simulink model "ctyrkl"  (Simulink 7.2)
settings: Solver=ode45  StartTime=0.0  StopTime=10.0  MaxStep=0.05  RelTol=1e-3
InitFcn:
  | init_ctyrkloub;
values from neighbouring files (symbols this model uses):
  L1 = 3    [init_ctyrkloub.m]    (also in init_klik.m = 1.5; init_withworth.m = 2)
  L2 = 5    [init_ctyrkloub.m]    (also in init_klik.m = v/sin(uhel3); init_withworth.m)
  L3 = 0.5    [init_ctyrkloub.m]    (also in init_klik.m = L1/(sin(uhel1)))
  L4 = 1    [init_ctyrkloub.m]
  omega = 1    [init_ctyrkloub.m]    (also in init_klik.m = 5; init_withworth.m = 0.5)
undefined symbols (not defined in the file or in its folder): deg, kg, m, N, rad, s
libraries: mblibv1 x17, simulink x3

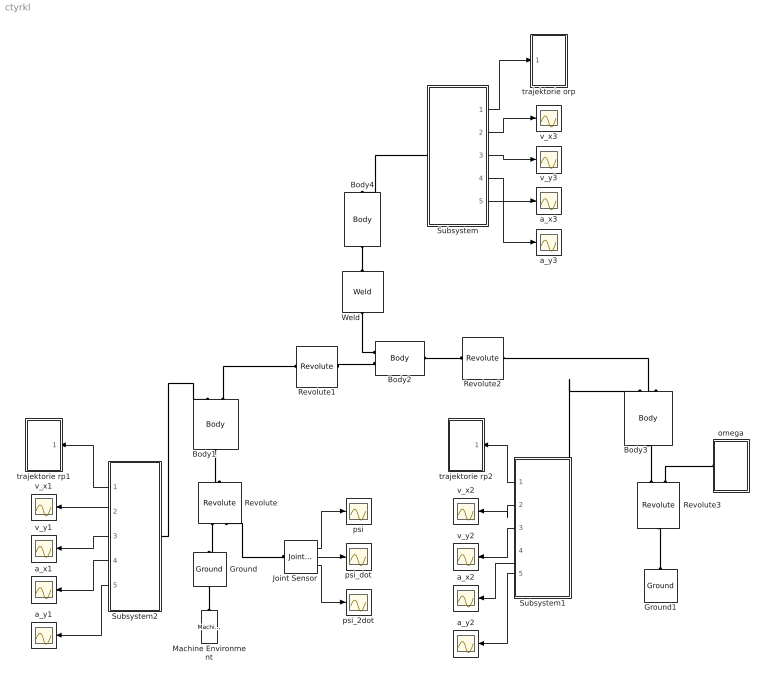
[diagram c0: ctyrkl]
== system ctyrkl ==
  Body1 : mblibv1/Bodies/Body  Orientation=up  DialogController=MECH.DynMechDlgSource  PhysicalDomain=mechanical  SubClassName=Unknown  LeftPortType=workingframe  RightPortType=workingframe  LConnTagsString=CS1  RConnTagsString=CS3|CS2  UpdateFromCAD=off  DialogClass=MechanicalBodyBlock  Mass=1  MassUnits=kg  InertiaUnits=kg*m^2  Inertia=eye(3)  Shape=Cylinder  ShapeDims=[1 1]  ShapeUnits=m  ShapeUse=false  Density=1  DensityUnits=kg/m^3  DensityUse=false  GraphicsMode=MACHINE_DEFAULT  BodyColorSelMode=MACHINE_DEFAULT  BodyColor=[1 0 0]  AttachedToCS=CG  CG=Left$CG$[L1*cos(pi/3) L1*sin(pi/3) 0]/2$CS1$CS1$m$[0 0 0]$Euler X-Y-Z$deg$WORLD$false$none  WorkingFrames=Right$CS3$[0 0 0]$CS2$CS2$m$[0 0 0]$Euler X-Y-Z$deg$WORLD$true$none#Left$CS1$[0 0 0]$Adjoining$Adjoining$m$[0 0 0]$Euler X-Y-Z$deg$WORLD$true$none#Right$CS2$[L1*cos(pi/3) L1*sin(pi/3) 0]$CS1$CS1$m$[0 0 0]$Euler X-Y-Z$deg$WORLD$true$none  CGPos=[L1*cos(pi/3) L1*sin(pi/3) 0]/2  CGRot=[0 0 0]  CS0Pos=[]  CS0Rot=[]  CS1Pos=[0 0 0]  CS1Rot=[0 0 0]  CS2Pos=[L1*cos(pi/3) L1*sin(pi/3) 0]  CS2Rot=[0 0 0]  CS3Pos=[0 0 0]  CS3Rot=[0 0 0]  CS4Pos=[]  CS4Rot=[]  CS5Pos=[]  CS5Rot=[]  CS6Pos=[]  CS6Rot=[]  CS7Pos=[]  CS7Rot=[]  CS8Pos=[]  CS8Rot=[]  CS9Pos=[]  CS9Rot=[]  CS10Pos=[]  CS10Rot=[]  CS11Pos=[]  CS11Rot=[]  CS12Pos=[]  CS12Rot=[]  CS13Pos=[]  CS13Rot=[]  CS14Pos=[]  CS14Rot=[]  CS15Pos=[]  CS15Rot=[]  CS16Pos=[]  CS16Rot=[]  CS17Pos=[]  CS17Rot=[]  CS18Pos=[]  CS18Rot=[]  CS19Pos=[]  CS19Rot=[]  CS20Pos=[]  CS20Rot=[]
  Body2 : mblibv1/Bodies/Body  DialogController=MECH.DynMechDlgSource  PhysicalDomain=mechanical  SubClassName=Unknown  LeftPortType=workingframe  RightPortType=workingframe  LConnTagsString=CG|CS1  RConnTagsString=CS2  UpdateFromCAD=off  DialogClass=MechanicalBodyBlock  Mass=1  MassUnits=kg  InertiaUnits=kg*m^2  Inertia=eye(3)  Shape=Cylinder  ShapeDims=[1 1]  ShapeUnits=m  ShapeUse=false  Density=1  DensityUnits=kg/m^3  DensityUse=false  GraphicsMode=MACHINE_DEFAULT  BodyColorSelMode=MACHINE_DEFAULT  BodyColor=[1 0 0]  AttachedToCS=CG  CG=Left$CG$[L2*cos(pi/6) -L2*sin(pi/6) 0]/2$CS1$CS1$m$[0 0 0]$Euler X-Y-Z$deg$WORLD$true$none  WorkingFrames=Left$CS1$[0 0 0]$Adjoining$Adjoining$m$[0 0 0]$Euler X-Y-Z$deg$WORLD$true$none#Right$CS2$[L2*cos(pi/6) -L2*sin(pi/6) 0]$CS1$CS1$m$[0 0 0]$Euler X-Y-Z$deg$WORLD$true$none  CGPos=[L2*cos(pi/6) -L2*sin(pi/6) 0]/2  CGRot=[0 0 0]  CS0Pos=[]  CS0Rot=[]  CS1Pos=[0 0 0]  CS1Rot=[0 0 0]  CS2Pos=[L2*cos(pi/6) -L2*sin(pi/6) 0]  CS2Rot=[0 0 0]  CS3Pos=[]  CS3Rot=[]  CS4Pos=[]  CS4Rot=[]  CS5Pos=[]  CS5Rot=[]  CS6Pos=[]  CS6Rot=[]  CS7Pos=[]  CS7Rot=[]  CS8Pos=[]  CS8Rot=[]  CS9Pos=[]  CS9Rot=[]  CS10Pos=[]  CS10Rot=[]  CS11Pos=[]  CS11Rot=[]  CS12Pos=[]  CS12Rot=[]  CS13Pos=[]  CS13Rot=[]  CS14Pos=[]  CS14Rot=[]  CS15Pos=[]  CS15Rot=[]  CS16Pos=[]  CS16Rot=[]  CS17Pos=[]  CS17Rot=[]  CS18Pos=[]  CS18Rot=[]  CS19Pos=[]  CS19Rot=[]  CS20Pos=[]  CS20Rot=[]
  Body3 : mblibv1/Bodies/Body  Orientation=down  DialogController=MECH.DynMechDlgSource  PhysicalDomain=mechanical  SubClassName=Unknown  LeftPortType=workingframe  RightPortType=workingframe  LConnTagsString=CS3|CS1  RConnTagsString=CS2  UpdateFromCAD=off  DialogClass=MechanicalBodyBlock  Mass=1  MassUnits=kg  InertiaUnits=kg*m^2  Inertia=eye(3)  Shape=Cylinder  ShapeDims=[1 1]  ShapeUnits=m  ShapeUse=false  Density=1  DensityUnits=kg/m^3  DensityUse=false  GraphicsMode=MACHINE_DEFAULT  BodyColorSelMode=MACHINE_DEFAULT  BodyColor=[1 0 0]  AttachedToCS=CG  CG=Left$CG$[L3*sin(pi/4) -L3*cos(pi/4) 0]/2$CS1$CS1$m$[0 0 0]$Euler X-Y-Z$deg$WORLD$false$none  WorkingFrames=Left$CS3$[0 0 0]$CS1$CS1$m$[0 0 0]$Euler X-Y-Z$deg$WORLD$true$none#Left$CS1$[0 0 0]$Adjoining$Adjoining$m$[0 0 0]$Euler X-Y-Z$deg$WORLD$true$none#Right$CS2$[L3*sin(pi/4) -L3*cos(pi/4) 0]$CS1$CS1$m$[0 0 0]$Euler X-Y-Z$deg$WORLD$true$none  CGPos=[L3*sin(pi/4) -L3*cos(pi/4) 0]/2  CGRot=[0 0 0]  CS0Pos=[]  CS0Rot=[]  CS1Pos=[0 0 0]  CS1Rot=[0 0 0]  CS2Pos=[L3*sin(pi/4) -L3*cos(pi/4) 0]  CS2Rot=[0 0 0]  CS3Pos=[0 0 0]  CS3Rot=[0 0 0]  CS4Pos=[]  CS4Rot=[]  CS5Pos=[]  CS5Rot=[]  CS6Pos=[]  CS6Rot=[]  CS7Pos=[]  CS7Rot=[]  CS8Pos=[]  CS8Rot=[]  CS9Pos=[]  CS9Rot=[]  CS10Pos=[]  CS10Rot=[]  CS11Pos=[]  CS11Rot=[]  CS12Pos=[]  CS12Rot=[]  CS13Pos=[]  CS13Rot=[]  CS14Pos=[]  CS14Rot=[]  CS15Pos=[]  CS15Rot=[]  CS16Pos=[]  CS16Rot=[]  CS17Pos=[]  CS17Rot=[]  CS18Pos=[]  CS18Rot=[]  CS19Pos=[]  CS19Rot=[]  CS20Pos=[]  CS20Rot=[]
  Body4 : mblibv1/Bodies/Body  Orientation=up  DialogController=MECH.DynMechDlgSource  PhysicalDomain=mechanical  SubClassName=Unknown  LeftPortType=workingframe  RightPortType=workingframe  LConnTagsString=CS1  RConnTagsString=CS2  UpdateFromCAD=off  DialogClass=MechanicalBodyBlock  Mass=1  MassUnits=kg  InertiaUnits=kg*m^2  Inertia=eye(3)  Shape=Cylinder  ShapeDims=[1 1]  ShapeUnits=m  ShapeUse=false  Density=1  DensityUnits=kg/m^3  DensityUse=false  GraphicsMode=MACHINE_DEFAULT  BodyColorSelMode=MACHINE_DEFAULT  BodyColor=[1 0 0]  AttachedToCS=CG  CG=Left$CG$[0 L4 0]/2$CS1$CS1$m$[0 0 0]$Euler X-Y-Z$deg$WORLD$false$none  WorkingFrames=Left$CS1$[0 0 0]$Adjoining$Adjoining$m$[0 0 0]$Euler X-Y-Z$deg$WORLD$true$none#Right$CS2$[0 L4 0]$CS1$CS1$m$[0 0 0]$Euler X-Y-Z$deg$WORLD$true$none  CGPos=[0 L4 0]/2  CGRot=[0 0 0]  CS0Pos=[]  CS0Rot=[]  CS1Pos=[0 0 0]  CS1Rot=[0 0 0]  CS2Pos=[0 L4 0]  CS2Rot=[0 0 0]  CS3Pos=[]  CS3Rot=[]  CS4Pos=[]  CS4Rot=[]  CS5Pos=[]  CS5Rot=[]  CS6Pos=[]  CS6Rot=[]  CS7Pos=[]  CS7Rot=[]  CS8Pos=[]  CS8Rot=[]  CS9Pos=[]  CS9Rot=[]  CS10Pos=[]  CS10Rot=[]  CS11Pos=[]  CS11Rot=[]  CS12Pos=[]  CS12Rot=[]  CS13Pos=[]  CS13Rot=[]  CS14Pos=[]  CS14Rot=[]  CS15Pos=[]  CS15Rot=[]  CS16Pos=[]  CS16Rot=[]  CS17Pos=[]  CS17Rot=[]  CS18Pos=[]  CS18Rot=[]  CS19Pos=[]  CS19Rot=[]  CS20Pos=[]  CS20Rot=[]
  Ground : mblibv1/Bodies/Ground  Orientation=up  DialogController=MECH.DynMechDlgSource  SystemSampleTime=-1  UpdateFromCAD=off  LeftPortType=env  RightPortType=workingframe  PhysicalDomain=Mechanical  DialogClass=GroundBlock  CoordPosition=[0 0 0]  CoordPositionUnits=m  StateVectorMgrId=0  MachineId=[1 0]  ShowEnvPort=on
  Ground1 : mblibv1/Bodies/Ground  Orientation=up  DialogController=MECH.DynMechDlgSource  SystemSampleTime=-1  UpdateFromCAD=off  LeftPortType=env  RightPortType=workingframe  PhysicalDomain=Mechanical  DialogClass=GroundBlock  CoordPosition=[L1*cos(pi/3)+L2*cos(pi/6)+L3*sin(pi/4) L1*sin(pi/3)-L2*sin(pi/6)-L3*cos(pi/4) 0]  CoordPositionUnits=m  StateVectorMgrId=-1  MachineId=[0 0]  ShowEnvPort=off
  Joint Sensor : mblibv1/Sensors &  Actuators/Joint Sensor  DialogController=MECH.DynMechDlgSource  SystemSampleTime=-1  UpdateFromCAD=off  PhysicalDomain=Mechanical  PortType=blob  Muxed=off  Pose=off  Angle=on  AngleUnits=rad  ArcVelocity=on  ArcVelocityUnits=rad/s  ArcAcceleration=on  ArcAccelerationUnits=rad/s^2  CoordPosition=on  CoordPositionUnits=m  Velocity=off  VelocityUnits=m/s  Acceleration=off  AccelerationUnits=m/s^2  Quaternion=on  QuaternionDT=off  QuaternionDDT=off  QuaternionUnits=off  OutputVector=[1]  ActiveIO=on  Width=3  DialogClass=MechanicalSensorBlock  Primitive=R1  Force=off  ForceUnits=N  Torque=off  TorqueUnits=N*m  ReferenceFrame=Absolute (World)  ReactionSensedSide=Base  ReactionReferenceFrame=Absolute (World)  ReactionForce=off  ReactionForceUnits=N  ReactionMoment=off  ReactionMomentUnits=N*m
  Machine Environment : mblibv1/Bodies/Machine Environment  Orientation=up  DialogController=MECH.DialogSource  SystemSampleTime=-1  PortType=env  PhysicalDomain=Mechanical  DialogTemplateClass=MECH.MachineEnvironment  SyncWhenCopied=off  Gravity=[0 -9.81 0]  GravityUnits=m/s^2  GravityAsSignal=off  Dimensionality=Auto-detect  AnalysisType=Kinematics  LinearAssemblyTolerance=1e-3  LinearAssemblyToleranceUnits=m  AngularAssemblyTolerance=1e-3  AngularAssemblyToleranceUnits=rad  ConstraintSolverType=Stabilizing  ConstraintRelTolerance=1e-4  ConstraintAbsTolerance=1e-4  UseRobustSingularityHandling=off  RedundancyAnalysisToleranceType=Automatically select tolerance  RedundancyAnalysisTolerance=1e-14  StatePerturbationType=Fixed  PerturbationSize=1e-5  VisualizeMachine=on  BodyVisualizationType=Use model default body geometries  BodyColorSelMode=Use model default  DefaultBodyColor=[1 0 0]
  Revolute : mblibv1/Joints/Revolute  Orientation=up  DialogController=MECH.DynMechDlgSource  PhysicalDomain=mechanical  SubClassName=Unknown  LeftPortType=blob  RightPortType=blob  LConnTagsString=__newl0|SA1  RConnTagsString=__newr0  UpdateFromCAD=off  NumSAPorts=1  CutJoint=off  MarkAsCut=off  Primitives=prismatic  PrimitiveProps=R1$World$[0 0 1]$revolute  DialogClass=JointBlock  R1Axis=[0 0 1]
  Revolute1 : mblibv1/Joints/Revolute  DialogController=MECH.DynMechDlgSource  PhysicalDomain=mechanical  SubClassName=Unknown  LeftPortType=blob  RightPortType=blob  LConnTagsString=__newl0  RConnTagsString=__newr0  UpdateFromCAD=off  NumSAPorts=0  CutJoint=off  MarkAsCut=off  Primitives=prismatic  PrimitiveProps=R1$WORLD$[0 0 1]$revolute  DialogClass=JointBlock  R1Axis=[0 0 1]
  Revolute2 : mblibv1/Joints/Revolute  DialogController=MECH.DynMechDlgSource  PhysicalDomain=mechanical  SubClassName=Unknown  LeftPortType=blob  RightPortType=blob  LConnTagsString=__newl0  RConnTagsString=__newr0  UpdateFromCAD=off  NumSAPorts=0  CutJoint=off  MarkAsCut=off  Primitives=prismatic  PrimitiveProps=R1$WORLD$[0 0 1]$revolute  DialogClass=JointBlock  R1Axis=[0 0 1]
  Revolute3 : mblibv1/Joints/Revolute  Orientation=down  DialogController=MECH.DynMechDlgSource  PhysicalDomain=mechanical  SubClassName=Unknown  LeftPortType=blob  RightPortType=blob  LConnTagsString=__newl0|SA1  RConnTagsString=__newr0  UpdateFromCAD=off  NumSAPorts=1  CutJoint=off  MarkAsCut=off  Primitives=prismatic  PrimitiveProps=R1$World$[0 0 1]$revolute  DialogClass=JointBlock  R1Axis=[0 0 1]
  Subsystem : Subsystem
  Subsystem1 : Subsystem  Orientation=left
  Subsystem2 : Subsystem  Orientation=left
  Weld : mblibv1/Joints/Weld  Orientation=up  DialogController=MECH.DynMechDlgSource  PhysicalDomain=mechanical  SubClassName=Unknown  LeftPortType=blob  RightPortType=blob  LConnTagsString=__newl0  RConnTagsString=__newr0  UpdateFromCAD=off  NumSAPorts=0  CutJoint=off  MarkAsCut=off  Primitives=weld  PrimitiveProps=W$WORLD$[0 0 0]$weld  DialogClass=JointBlock  WAxis=[0 0 0]
  a_x1 : Scope
  a_x2 : Scope
  a_x3 : Scope
  a_y1 : Scope
  a_y2 : Scope
  a_y3 : Scope
  omega : Subsystem  Orientation=left
  psi : Scope
  psi_2dot : Scope
  psi_dot : Scope
  trajektorie orp : Subsystem
  trajektorie rp1 : Subsystem  Orientation=left
  trajektorie rp2 : Subsystem  Orientation=left
  v_x1 : Scope
  v_x2 : Scope
  v_x3 : Scope
  v_y1 : Scope
  v_y2 : Scope
  v_y3 : Scope
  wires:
  Subsystem/1(Out1) -> trajektorie orp/1(In1)
  Subsystem/2(Out2) -> v_x3/1
  Subsystem/3(Out3) -> v_y3/1
  Subsystem/4(Out4) -> a_x3/1
  Subsystem/5(Out5) -> a_y3/1
  Subsystem1/1(Out1) -> trajektorie rp2/1(In1)
  Subsystem1/2(Out2) -> v_x2/1
  Subsystem1/3(Out3) -> v_y2/1
  Subsystem1/4(Out4) -> a_x2/1
  Subsystem1/5(Out5) -> a_y2/1
  Subsystem2/1(Out1) -> trajektorie rp1/1(In1)
  Subsystem2/2(Out2) -> v_x1/1
  Subsystem2/3(Out3) -> v_y1/1
  Subsystem2/4(Out4) -> a_x1/1
  Subsystem2/5(Out5) -> a_y1/1
  Joint Sensor/1 -> psi/1
  Joint Sensor/2 -> psi_dot/1
  Joint Sensor/3 -> psi_2dot/1
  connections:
  Machine Environment/RConn1 -- Ground/LConn1
  Revolute/LConn1 -- Ground/RConn1
  Body1/LConn1 -- Revolute/RConn1
  Revolute1/RConn1 -- Body2/LConn2
  Revolute2/LConn1 -- Body2/RConn1
  Revolute3/LConn1 -- Body3/RConn1
  Ground1/RConn1 -- Revolute3/RConn1
  Weld/LConn1 -- Body2/LConn1
  Body4/LConn1 -- Weld/RConn1
  Body1/RConn2 -- Revolute1/LConn1
  Revolute3/LConn2 -- omega/RConn1
  Revolute2/RConn1 -- Body3/LConn2
  Subsystem1/LConn1 -- Body3/LConn1
  Subsystem/LConn1 -- Body4/RConn1
  Subsystem2/LConn1 -- Body1/RConn1
  Joint Sensor/LConn1 -- Revolute/LConn2

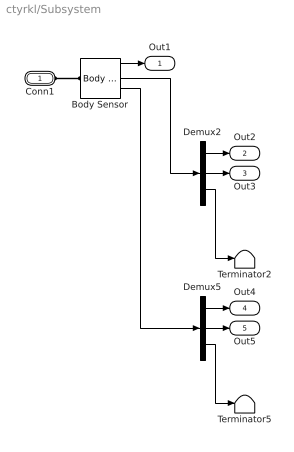
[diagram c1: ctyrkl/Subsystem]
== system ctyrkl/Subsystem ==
  Body Sensor : mblibv1/Sensors &  Actuators/Body Sensor  DialogController=MECH.DynMechDlgSource  SystemSampleTime=-1  UpdateFromCAD=off  PhysicalDomain=Mechanical  PortType=blob  Muxed=off  Pose=off  Angle=on  AngleUnits=deg  ArcVelocity=off  ArcVelocityUnits=deg/s  ArcAcceleration=off  ArcAccelerationUnits=deg/s^2  CoordPosition=on  CoordPositionUnits=m  Velocity=on  VelocityUnits=m/s  Acceleration=on  AccelerationUnits=m/s^2  Quaternion=on  QuaternionDT=off  QuaternionDDT=off  QuaternionUnits=off  OutputVector=[1]  ActiveIO=on  Width=9  DialogClass=MechanicalSensorBlock  ReferenceFrame=Absolute (World)
  Demux2 : Demux  Outputs=3
  Demux5 : Demux  Outputs=3
  Terminator2 : Terminator
  Terminator5 : Terminator
  Conn1 : PMIOPort  Port=1  Side=Left
  Out1 : Outport
  Out2 : Outport  Port=2
  Out3 : Outport  Port=3
  Out4 : Outport  Port=4
  Out5 : Outport  Port=5
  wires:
  Demux2/3 -> Terminator2/1
  Body Sensor/2 -> Demux2/1
  Demux5/3 -> Terminator5/1
  Body Sensor/3 -> Demux5/1
  Body Sensor/1 -> Out1/1
  Demux2/1 -> Out2/1
  Demux2/2 -> Out3/1
  Demux5/1 -> Out4/1
  Demux5/2 -> Out5/1
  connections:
  Conn1/RConn1 -- Body Sensor/LConn1

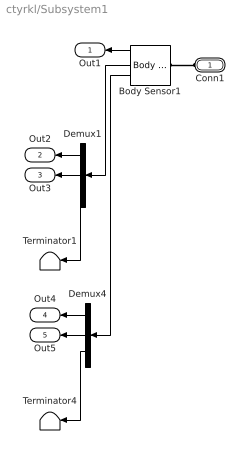
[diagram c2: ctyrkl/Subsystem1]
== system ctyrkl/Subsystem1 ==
  Body Sensor1 : mblibv1/Sensors &  Actuators/Body Sensor  Orientation=left  DialogController=MECH.DynMechDlgSource  SystemSampleTime=-1  UpdateFromCAD=off  PhysicalDomain=Mechanical  PortType=blob  Muxed=off  Pose=off  Angle=on  AngleUnits=deg  ArcVelocity=off  ArcVelocityUnits=deg/s  ArcAcceleration=off  ArcAccelerationUnits=deg/s^2  CoordPosition=on  CoordPositionUnits=m  Velocity=on  VelocityUnits=m/s  Acceleration=on  AccelerationUnits=m/s^2  Quaternion=on  QuaternionDT=off  QuaternionDDT=off  QuaternionUnits=off  OutputVector=[1]  ActiveIO=on  Width=9  DialogClass=MechanicalSensorBlock  ReferenceFrame=Absolute (World)
  Demux1 : Demux  Orientation=left  Outputs=3
  Demux4 : Demux  Orientation=left  Outputs=3
  Terminator1 : Terminator
  Terminator4 : Terminator
  Conn1 : PMIOPort  Orientation=left  Port=1  Side=Left
  Out1 : Outport  Orientation=left
  Out2 : Outport  Orientation=left  Port=2
  Out3 : Outport  Orientation=left  Port=3
  Out4 : Outport  Orientation=left  Port=4
  Out5 : Outport  Orientation=left  Port=5
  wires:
  Demux1/3 -> Terminator1/1
  Body Sensor1/2 -> Demux1/1
  Demux4/3 -> Terminator4/1
  Body Sensor1/3 -> Demux4/1
  Body Sensor1/1 -> Out1/1
  Demux1/1 -> Out2/1
  Demux1/2 -> Out3/1
  Demux4/1 -> Out4/1
  Demux4/2 -> Out5/1
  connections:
  Conn1/RConn1 -- Body Sensor1/LConn1

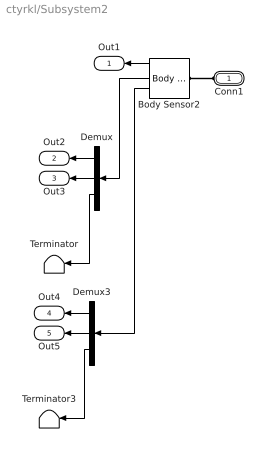
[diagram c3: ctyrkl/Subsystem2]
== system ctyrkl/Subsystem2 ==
  Body Sensor2 : mblibv1/Sensors &  Actuators/Body Sensor  Orientation=left  DialogController=MECH.DynMechDlgSource  SystemSampleTime=-1  UpdateFromCAD=off  PhysicalDomain=Mechanical  PortType=blob  Muxed=off  Pose=off  Angle=on  AngleUnits=deg  ArcVelocity=off  ArcVelocityUnits=deg/s  ArcAcceleration=off  ArcAccelerationUnits=deg/s^2  CoordPosition=on  CoordPositionUnits=m  Velocity=on  VelocityUnits=m/s  Acceleration=on  AccelerationUnits=m/s^2  Quaternion=on  QuaternionDT=off  QuaternionDDT=off  QuaternionUnits=off  OutputVector=[1]  ActiveIO=on  Width=9  DialogClass=MechanicalSensorBlock  ReferenceFrame=Absolute (World)
  Demux : Demux  Orientation=left  Outputs=3
  Demux3 : Demux  Orientation=left  Outputs=3
  Terminator : Terminator
  Terminator3 : Terminator
  Conn1 : PMIOPort  Orientation=left  Port=1  Side=Left
  Out1 : Outport  Orientation=left
  Out2 : Outport  Orientation=left  Port=2
  Out3 : Outport  Orientation=left  Port=3
  Out4 : Outport  Orientation=left  Port=4
  Out5 : Outport  Orientation=left  Port=5
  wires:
  Body Sensor2/2 -> Demux/1
  Demux/3 -> Terminator/1
  Demux3/3 -> Terminator3/1
  Body Sensor2/3 -> Demux3/1
  Body Sensor2/1 -> Out1/1
  Demux/1 -> Out2/1
  Demux/2 -> Out3/1
  Demux3/1 -> Out4/1
  Demux3/2 -> Out5/1
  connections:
  Conn1/RConn1 -- Body Sensor2/LConn1

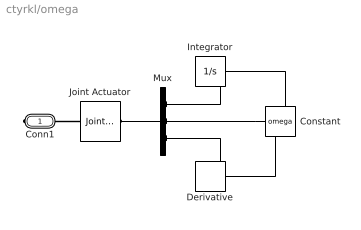
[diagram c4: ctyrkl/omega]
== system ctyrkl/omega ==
  Constant : Constant  Value=omega  OutDataType=sfix(16)  OutScaling=2^0
  Derivative : Derivative
  Integrator : Integrator
  Joint Actuator : mblibv1/Sensors &  Actuators/Joint Actuator  DialogController=MECH.DynMechDlgSource  SystemSampleTime=-1  UpdateFromCAD=off  PhysicalDomain=Mechanical  PortType=blob  ActuationStyle=Motion  AngleUnits=rad  ArcVelocityUnits=rad/s  ArcAccelerationUnits=rad/s^2  CoordPositionUnits=m  VelocityUnits=m/s  AccelerationUnits=m/s^2  ForceUnits=N  TorqueUnits=N*m  ActiveIO=on  Width=3  DialogClass=MechanicalActuatorBlock  Primitive=R1  ReferenceFrame=Absolute (World)
  Mux : Mux  Inputs=3
  Conn1 : PMIOPort  Port=1  Side=Right
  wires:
  Constant/1 -> Mux/2, Derivative/1, Integrator/1
  Derivative/1 -> Mux/3
  Integrator/1 -> Mux/1
  Mux/1 -> Joint Actuator/1
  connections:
  Conn1/RConn1 -- Joint Actuator/RConn1

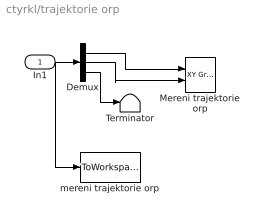
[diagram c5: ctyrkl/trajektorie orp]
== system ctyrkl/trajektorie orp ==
  In1 : Inport
  Demux : Demux  Outputs=3
  Mereni trajektorie orp : simulink/Sinks/XY Graph  SystemSampleTime=-1  xmin=3.6  xmax=4.5  ymin=1.4  ymax=2.6  st=-1
  Terminator : Terminator
  mereni trajektorie orp : ToWorkspace  VariableName=orp  SampleTime=-1  SaveFormat=Array
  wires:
  Demux/1 -> Mereni trajektorie orp/1
  Demux/2 -> Mereni trajektorie orp/2
  Demux/3 -> Terminator/1
  In1/1 -> Demux/1, mereni trajektorie orp/1

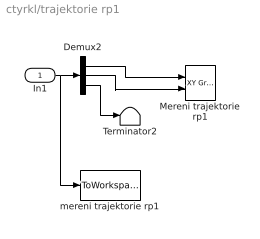
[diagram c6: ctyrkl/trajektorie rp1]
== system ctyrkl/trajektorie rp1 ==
  In1 : Inport
  Demux2 : Demux  Outputs=3
  Mereni trajektorie rp1 : simulink/Sinks/XY Graph  SystemSampleTime=-1  xmin=1  xmax=3  ymin=1.5  ymax=3  st=-1
  Terminator2 : Terminator
  mereni trajektorie rp1 : ToWorkspace  VariableName=rot1  SampleTime=-1  SaveFormat=Array
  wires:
  Demux2/1 -> Mereni trajektorie rp1/1
  Demux2/2 -> Mereni trajektorie rp1/2
  Demux2/3 -> Terminator2/1
  In1/1 -> Demux2/1, mereni trajektorie rp1/1

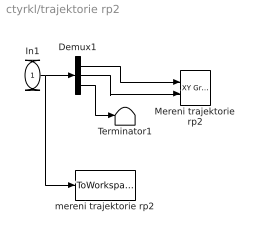
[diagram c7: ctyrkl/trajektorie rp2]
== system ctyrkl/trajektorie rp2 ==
  In1 : Inport
  Demux1 : Demux  Outputs=3
  Mereni trajektorie rp2 : simulink/Sinks/XY Graph  SystemSampleTime=-1  xmin=5  xmax=7  ymin=-1  ymax=0.5  st=-1
  Terminator1 : Terminator
  mereni trajektorie rp2 : ToWorkspace  VariableName=rot  SampleTime=-1  SaveFormat=Array
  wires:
  Demux1/1 -> Mereni trajektorie rp2/1
  Demux1/2 -> Mereni trajektorie rp2/2
  Demux1/3 -> Terminator1/1
  In1/1 -> Demux1/1, mereni trajektorie rp2/1
